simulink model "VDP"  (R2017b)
settings: Solver=FixedStepDiscrete  StartTime=0.0  StopTime=10.0  FixedStep=0.01  RelTol=1e-3  EnableMultiTasking=on
undefined symbols (not defined in the file): ASWTYPE_FALSE, ASWTYPE_TRUE, CcVDP_DiagPermitDelayTi_ms, CcVDP_LeadAcidChgHvOnTi_ms, Enum_ISPNetWkUpSt, VDP0B5_RUNTIME_MS, VDP2A3_RUNTIME_MS, VDP_CONST18000_NUMB, VDP_CONST2080_NUMB, VDP_CONST6000_NUMB
libraries: AIWAYS_Powertrain_BMS_lib x35

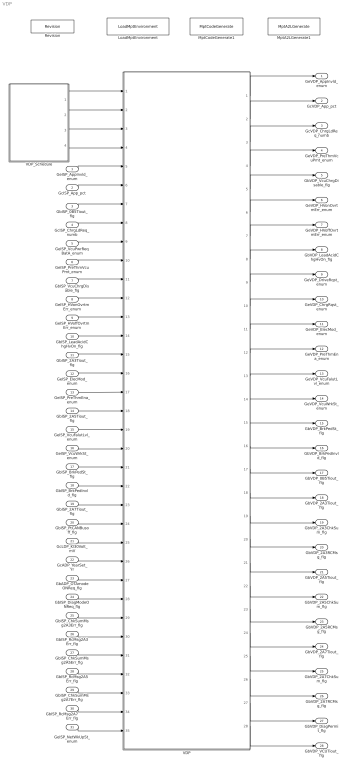
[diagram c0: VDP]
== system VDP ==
  GeISP_AppInvld_enum : Inport
  GcISP_App_pct : Inport  Port=2
  GbISP_0B5Tiout_flg : Inport  Port=3
  GcISP_ChrgLdReq_numb : Inport  Port=4
  GeISP_VcuPwrReqBatA_enum : Inport  Port=5
  GeISP_PreThmVcuPmt_enum : Inport  Port=6
  GbISP_VcuChrgDisable_flg : Inport  Port=7
  GeISP_HVonOvrtmErr_enum : Inport  Port=8
  GeISP_HVoffOvrtmErr_enum : Inport  Port=9
  GbISP_LeadAcidChgHvOn_flg : Inport  Port=10
  GbISP_2A3Tiout_flg : Inport  Port=11
  GeISP_ElecMod_enum : Inport  Port=12
  GeISP_PreThmEna_enum : Inport  Port=13
  GbISP_2A5Tiout_flg : Inport  Port=14
  GeISP_VcuFalutLvl_enum : Inport  Port=15
  GeISP_VcuWrkSt_enum : Inport  Port=16
  GbISP_BrkPedSt_flg : Inport  Port=17
  GbISP_BrkPedInvld_flg : Inport  Port=18
  GbISP_2A7Tiout_flg : Inport  Port=19
  GbISP_PtCANBusoff_flg : Inport  Port=20
  GcLDP_Kl30Volt_mV : Inport  Port=21
  GcADP_YearSet_Yr : Inport  Port=22
  GbADP_OTAmodeONReq_flg : Inport  Port=23
  GbISP_DiagModeONReq_flg : Inport  Port=24
  GbISP_ChkSumMsg2A3Err_flg : Inport  Port=25
  GbISP_RcMsg2A3Err_flg : Inport  Port=26
  GbISP_ChkSumMsg2A5Err_flg : Inport  Port=27
  GbISP_RcMsg2A5Err_flg : Inport  Port=28
  GbISP_ChkSumMsg2A7Err_flg : Inport  Port=29
  GbISP_RcMsg2A7Err_flg : Inport  Port=30
  GeISP_NetWkUpSt_enum : Inport  Port=31
  LoadMptEnvironment : AIWAYS_Powertrain_BMS_lib/Config/LoadMptEnvironment  ProjectName=Comm  SuppierID=NewPlatformUAES
  MptA2LGenerate1 : AIWAYS_Powertrain_BMS_lib/Config/MptA2LGenerate  SystemSampleTime=-1
  MptCodeGenerate1 : AIWAYS_Powertrain_BMS_lib/Config/MptCodeGenerate  SystemSampleTime=-1
  Revision : AIWAYS_Powertrain_BMS_lib/Config/Revision  curVersion='M104C104'  newVersion='M104C104'
  VDP : Subsystem
  VDP_Schedule : Stateflow chart  TreatAsAtomicUnit=on
  GeVDP_AppInvld_enum : Outport
  GcVDP_App_pct : Outport  Port=2
  GcVDP_ChrgLdReq_numb : Outport  Port=3
  GeVDP_PreThmVcuPmt_enum : Outport  Port=4
  GbVDP_VcuChrgDisable_flg : Outport  Port=5
  GeVDP_HVonOvrtmErr_enum : Outport  Port=6
  GeVDP_HVoffOvrtmErr_enum : Outport  Port=7
  GbVDP_LeadAcidChgHvOn_flg : Outport  Port=8
  GeVDP_DriveRqst_enum : Outport  Port=9
  GeVDP_ChrgRqst_enum : Outport  Port=10
  GeVDP_ElecMod_enum : Outport  Port=11
  GeVDP_PreThmEna_enum : Outport  Port=12
  GeVDP_VcuFalutLvl_enum : Outport  Port=13
  GeVDP_VcuWrkSt_enum : Outport  Port=14
  GbVDP_BrkPedSt_flg : Outport  Port=15
  GbVDP_BrkPedInvld_flg : Outport  Port=16
  GbVDP_0B5Tiout_flg : Outport  Port=17
  GbVDP_2A3Tiout_flg : Outport  Port=18
  GbVDP_2A3ChkSum_flg : Outport  Port=19
  GbVDP_2A3RCMsg_flg : Outport  Port=20
  GbVDP_2A5Tiout_flg : Outport  Port=21
  GbVDP_2A5ChkSum_flg : Outport  Port=22
  GbVDP_2A5RCMsg_flg : Outport  Port=23
  GbVDP_2A7Tiout_flg : Outport  Port=24
  GbVDP_2A7ChkSum_flg : Outport  Port=25
  GbVDP_2A7RCMsg_flg : Outport  Port=26
  GbVDP_DiagPermit_flg : Outport  Port=27
  GbVDP_VCUTiout_flg : Outport  Port=28
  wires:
  GeISP_AppInvld_enum/1 -> VDP/5(GeISP_AppInvld_enum)
  GcISP_App_pct/1 -> VDP/6(GcISP_App_pct)
  GbISP_0B5Tiout_flg/1 -> VDP/7(GbISP_0B5Tiout_flg)
  GcISP_ChrgLdReq_numb/1 -> VDP/8(GcISP_ChrgLdReq_numb)
  GeISP_VcuPwrReqBatA_enum/1 -> VDP/9(GeISP_VcuPwrReqBatA_enum)
  GeISP_PreThmVcuPmt_enum/1 -> VDP/10(GeISP_PreThmVcuPmt_enum)
  GbISP_VcuChrgDisable_flg/1 -> VDP/11(GbISP_VcuChrgDisable_flg)
  GeISP_HVonOvrtmErr_enum/1 -> VDP/12(GeISP_HVonOvrtmErr_enum)
  GeISP_HVoffOvrtmErr_enum/1 -> VDP/13(GeISP_HVoffOvrtmErr_enum)
  GbISP_LeadAcidChgHvOn_flg/1 -> VDP/14(GbISP_LeadAcidChgHvOn_flg)
  GbISP_2A3Tiout_flg/1 -> VDP/15(GbISP_2A3Tiout_flg)
  GeISP_ElecMod_enum/1 -> VDP/16(GeISP_ElecMod_enum)
  GeISP_PreThmEna_enum/1 -> VDP/17(GeISP_PreThmEna_enum)
  GbISP_2A5Tiout_flg/1 -> VDP/18(GbISP_2A5Tiout_flg)
  GeISP_VcuFalutLvl_enum/1 -> VDP/19(GeISP_VcuFalutLvl_enum)
  GeISP_VcuWrkSt_enum/1 -> VDP/20(GeISP_VcuWrkSt_enum)
  GbISP_BrkPedSt_flg/1 -> VDP/21(GbISP_BrkPedSt_flg)
  GbISP_BrkPedInvld_flg/1 -> VDP/22(GbISP_BrkPedInvld_flg)
  GbISP_2A7Tiout_flg/1 -> VDP/23(GbISP_2A7Tiout_flg)
  VDP/1(GeVDP_AppInvld_enum) -> GeVDP_AppInvld_enum/1
  VDP/2(GcVDP_App_pct) -> GcVDP_App_pct/1
  VDP/3(GcVDP_ChrgLdReq_numb) -> GcVDP_ChrgLdReq_numb/1
  VDP/4(GeVDP_PreThmVcuPmt_enum) -> GeVDP_PreThmVcuPmt_enum/1
  VDP/5(GbVDP_VcuChrgDisable_flg) -> GbVDP_VcuChrgDisable_flg/1
  VDP/6(GeVDP_HVonOvrtmErr_enum) -> GeVDP_HVonOvrtmErr_enum/1
  VDP/7(GeVDP_HVoffOvrtmErr_enum) -> GeVDP_HVoffOvrtmErr_enum/1
  VDP/8(GbVDP_LeadAcidChgHvOn_flg) -> GbVDP_LeadAcidChgHvOn_flg/1
  VDP/9(GeVDP_DriveRqst_enum) -> GeVDP_DriveRqst_enum/1
  VDP/10(GeVDP_ChrgRqst_enum) -> GeVDP_ChrgRqst_enum/1
  VDP/11(GeVDP_ElecMod_enum) -> GeVDP_ElecMod_enum/1
  VDP/12(GeVDP_PreThmEna_enum) -> GeVDP_PreThmEna_enum/1
  VDP/13(GeVDP_VcuFalutLvl_enum) -> GeVDP_VcuFalutLvl_enum/1
  VDP/14(GeVDP_VcuWrkSt_enum) -> GeVDP_VcuWrkSt_enum/1
  VDP/15(GbVDP_BrkPedSt_flg) -> GbVDP_BrkPedSt_flg/1
  VDP/16(GbVDP_BrkPedInvld_flg) -> GbVDP_BrkPedInvld_flg/1
  GbISP_DiagModeONReq_flg/1 -> VDP/28(GbISP_DiagModeONReq_flg)
  GcLDP_Kl30Volt_mV/1 -> VDP/25(GcLDP_Kl30Volt_mV)
  GbADP_OTAmodeONReq_flg/1 -> VDP/27(GbADP_OTAmodeONReq_flg)
  GcADP_YearSet_Yr/1 -> VDP/26(GcADP_YearSet_Yr)
  GbISP_PtCANBusoff_flg/1 -> VDP/24(GbISP_PtCANBusoff_flg)
  GbISP_ChkSumMsg2A3Err_flg/1 -> VDP/29(GbISP_ChkSumMsg2A3Err_flg)
  GbISP_RcMsg2A3Err_flg/1 -> VDP/30(GbISP_RcMsg2A3Err_flg)
  GbISP_RcMsg2A5Err_flg/1 -> VDP/32(GbISP_RcMsg2A5Err_flg)
  GbISP_ChkSumMsg2A5Err_flg/1 -> VDP/31(GbISP_ChkSumMsg2A5Err_flg)
  GbISP_RcMsg2A7Err_flg/1 -> VDP/34(GbISP_RcMsg2A7Err_flg)
  GbISP_ChkSumMsg2A7Err_flg/1 -> VDP/33(GbISP_ChkSumMsg2A7Err_flg)
  VDP/17(GbVDP_0B5Tiout_flg) -> GbVDP_0B5Tiout_flg/1
  VDP/20(GbVDP_2A3RCMsg_flg) -> GbVDP_2A3RCMsg_flg/1
  VDP/18(GbVDP_2A3Tiout_flg) -> GbVDP_2A3Tiout_flg/1
  VDP/19(GbVDP_2A3ChkSum_flg) -> GbVDP_2A3ChkSum_flg/1
  VDP/23(GbVDP_2A5RCMsg_flg) -> GbVDP_2A5RCMsg_flg/1
  VDP/21(GbVDP_2A5Tiout_flg) -> GbVDP_2A5Tiout_flg/1
  VDP/22(GbVDP_2A5ChkSum_flg) -> GbVDP_2A5ChkSum_flg/1
  VDP/25(GbVDP_2A7ChkSum_flg) -> GbVDP_2A7ChkSum_flg/1
  VDP/24(GbVDP_2A7Tiout_flg) -> GbVDP_2A7Tiout_flg/1
  VDP/26(GbVDP_2A7RCMsg_flg) -> GbVDP_2A7RCMsg_flg/1
  VDP/27(GbVDP_DiagPermit_flg) -> GbVDP_DiagPermit_flg/1
  VDP/28(GbVDP_VCUTiout_flg) -> GbVDP_VCUTiout_flg/1
  GeISP_NetWkUpSt_enum/1 -> VDP/35(GeISP_NetWkUpSt_enum)
  VDP_Schedule/3(VDP_2A5_100ms()) -> VDP/3(VDP_2A5_100ms)
  VDP_Schedule/2(VDP_2A3_10ms()) -> VDP/2(VDP_2A3_10ms)
  VDP_Schedule/1(VDP_0B5_10ms()) -> VDP/1(VDP_0B5_10ms)
  VDP_Schedule/4(VDP_2A7_100ms()) -> VDP/4(VDP_2A7_100ms)

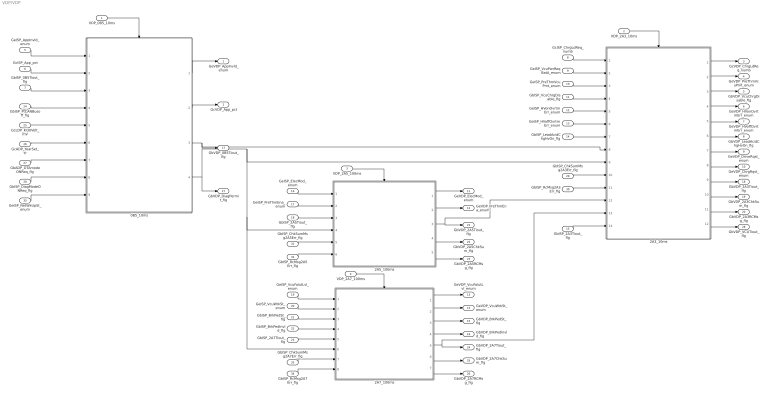
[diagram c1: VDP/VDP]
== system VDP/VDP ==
  VDP_0B5_10ms : Inport
  VDP_2A3_10ms : Inport  Port=2
  VDP_2A5_100ms : Inport  Port=3
  VDP_2A7_100ms : Inport  Port=4
  GeISP_AppInvld_enum : Inport  Port=5
  GcISP_App_pct : Inport  Port=6
  GbISP_0B5Tiout_flg : Inport  Port=7
  GcISP_ChrgLdReq_numb : Inport  Port=8
  GeISP_VcuPwrReqBatA_enum : Inport  Port=9
  GeISP_PreThmVcuPmt_enum : Inport  Port=10
  GbISP_VcuChrgDisable_flg : Inport  Port=11
  GeISP_HVonOvrtmErr_enum : Inport  Port=12
  GeISP_HVoffOvrtmErr_enum : Inport  Port=13
  GbISP_LeadAcidChgHvOn_flg : Inport  Port=14
  GbISP_2A3Tiout_flg : Inport  Port=15
  GeISP_ElecMod_enum : Inport  Port=16
  GeISP_PreThmEna_enum : Inport  Port=17
  GbISP_2A5Tiout_flg : Inport  Port=18
  GeISP_VcuFalutLvl_enum : Inport  Port=19
  GeISP_VcuWrkSt_enum : Inport  Port=20
  GbISP_BrkPedSt_flg : Inport  Port=21
  GbISP_BrkPedInvld_flg : Inport  Port=22
  GbISP_2A7Tiout_flg : Inport  Port=23
  GbISP_PtCANBusoff_flg : Inport  Port=24
  GcLDP_Kl30Volt_mV : Inport  Port=25
  GcADP_YearSet_Yr : Inport  Port=26
  GbADP_OTAmodeONReq_flg : Inport  Port=27
  GbISP_DiagModeONReq_flg : Inport  Port=28
  GbISP_ChkSumMsg2A3Err_flg : Inport  Port=29
  GbISP_RcMsg2A3Err_flg : Inport  Port=30
  GbISP_ChkSumMsg2A5Err_flg : Inport  Port=31
  GbISP_RcMsg2A5Err_flg : Inport  Port=32
  GbISP_ChkSumMsg2A7Err_flg : Inport  Port=33
  GbISP_RcMsg2A7Err_flg : Inport  Port=34
  GeISP_NetWkUpSt_enum : Inport  Port=35
  0B5_10ms : Subsystem
  2A3_10ms : Subsystem
  2A5_100ms : Subsystem
  2A7_100ms : Subsystem
  GeVDP_AppInvld_enum : Outport
  GcVDP_App_pct : Outport  Port=2
  GcVDP_ChrgLdReq_numb : Outport  Port=3
  GeVDP_PreThmVcuPmt_enum : Outport  Port=4
  GbVDP_VcuChrgDisable_flg : Outport  Port=5
  GeVDP_HVonOvrtmErr_enum : Outport  Port=6
  GeVDP_HVoffOvrtmErr_enum : Outport  Port=7
  GbVDP_LeadAcidChgHvOn_flg : Outport  Port=8
  GeVDP_DriveRqst_enum : Outport  Port=9
  GeVDP_ChrgRqst_enum : Outport  Port=10
  GeVDP_ElecMod_enum : Outport  Port=11
  GeVDP_PreThmEna_enum : Outport  Port=12
  GeVDP_VcuFalutLvl_enum : Outport  Port=13
  GeVDP_VcuWrkSt_enum : Outport  Port=14
  GbVDP_BrkPedSt_flg : Outport  Port=15
  GbVDP_BrkPedInvld_flg : Outport  Port=16
  GbVDP_0B5Tiout_flg : Outport  Port=17
  GbVDP_2A3Tiout_flg : Outport  Port=18
  GbVDP_2A3ChkSum_flg : Outport  Port=19
  GbVDP_2A3RCMsg_flg : Outport  Port=20
  GbVDP_2A5Tiout_flg : Outport  Port=21
  GbVDP_2A5ChkSum_flg : Outport  Port=22
  GbVDP_2A5RCMsg_flg : Outport  Port=23
  GbVDP_2A7Tiout_flg : Outport  Port=24
  GbVDP_2A7ChkSum_flg : Outport  Port=25
  GbVDP_2A7RCMsg_flg : Outport  Port=26
  GbVDP_DiagPermit_flg : Outport  Port=27
  GbVDP_VCUTiout_flg : Outport  Port=28
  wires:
  VDP_2A3_10ms/1 -> 2A3_10ms/Trigger
  VDP_2A5_100ms/1 -> 2A5_100ms/Trigger
  VDP_2A7_100ms/1 -> 2A7_100ms/Trigger
  GeISP_AppInvld_enum/1 -> 0B5_10ms/1(GeISP_AppInvld_enum)
  GcISP_App_pct/1 -> 0B5_10ms/2(GcISP_App_pct)
  GbISP_0B5Tiout_flg/1 -> 0B5_10ms/3(GbISP_0B5Tiout_flg)
  0B5_10ms/1(GeVDP_AppInvld_enum) -> GeVDP_AppInvld_enum/1
  0B5_10ms/2(GcVDP_App_pct) -> GcVDP_App_pct/1
  GcISP_ChrgLdReq_numb/1 -> 2A3_10ms/1(GcISP_ChrgLdReq_numb)
  GeISP_VcuPwrReqBatA_enum/1 -> 2A3_10ms/2(GeISP_VcuPwrReqBatA_enum)
  GeISP_PreThmVcuPmt_enum/1 -> 2A3_10ms/3(GeISP_PreThmVcuPmt_enum)
  GbISP_VcuChrgDisable_flg/1 -> 2A3_10ms/4(GbISP_VcuChrgDisable_flg)
  GeISP_HVonOvrtmErr_enum/1 -> 2A3_10ms/5(GeISP_HVonOvrtmErr_enum)
  GeISP_HVoffOvrtmErr_enum/1 -> 2A3_10ms/6(GeISP_HVoffOvrtmErr_enum)
  GbISP_LeadAcidChgHvOn_flg/1 -> 2A3_10ms/7(GbISP_LeadAcidChgHvOn_flg)
  GbISP_2A3Tiout_flg/1 -> 2A3_10ms/14(GbISP_2A3Tiout_flg)
  2A3_10ms/5(GeVDP_HVoffOvrtmErr_enum) -> GeVDP_HVoffOvrtmErr_enum/1
  2A3_10ms/4(GeVDP_HVonOvrtmErr_enum) -> GeVDP_HVonOvrtmErr_enum/1
  2A3_10ms/6(GbVDP_LeadAcidChgHvOn_flg) -> GbVDP_LeadAcidChgHvOn_flg/1
  2A3_10ms/3(GbVDP_VcuChrgDisable_flg) -> GbVDP_VcuChrgDisable_flg/1
  2A3_10ms/2(GeVDP_PreThmVcuPmt_enum) -> GeVDP_PreThmVcuPmt_enum/1
  2A3_10ms/1(GcVDP_ChrgLdReq_numb) -> GcVDP_ChrgLdReq_numb/1
  2A3_10ms/7(GeVDP_DriveRqst_enum) -> GeVDP_DriveRqst_enum/1
  2A3_10ms/8(GeVDP_ChrgRqst_enum) -> GeVDP_ChrgRqst_enum/1
  GeISP_ElecMod_enum/1 -> 2A5_100ms/1(GeISP_ElecMod_enum)
  GeISP_PreThmEna_enum/1 -> 2A5_100ms/2(GeISP_PreThmEna_enum)
  GbISP_2A5Tiout_flg/1 -> 2A5_100ms/3(GbISP_2A5Tiout_flg)
  2A5_100ms/1(GeVDP_ElecMod_enum) -> GeVDP_ElecMod_enum/1
  2A5_100ms/2(GeVDP_PreThmEna_enum) -> GeVDP_PreThmEna_enum/1
  GeISP_VcuFalutLvl_enum/1 -> 2A7_100ms/1(GeISP_VcuFalutLvl_enum)
  GeISP_VcuWrkSt_enum/1 -> 2A7_100ms/2(GeISP_VcuWrkSt_enum)
  GbISP_BrkPedSt_flg/1 -> 2A7_100ms/3(GbISP_BrkPedSt_flg)
  GbISP_BrkPedInvld_flg/1 -> 2A7_100ms/4(GbISP_BrkPedInvld_flg)
  GbISP_2A7Tiout_flg/1 -> 2A7_100ms/5(GbISP_2A7Tiout_flg)
  2A7_100ms/1(GeVDP_VcuFalutLvl_enum) -> GeVDP_VcuFalutLvl_enum/1
  2A7_100ms/2(GeVDP_VcuWrkSt_enum) -> GeVDP_VcuWrkSt_enum/1
  2A7_100ms/3(GbVDP_BrkPedSt_flg) -> GbVDP_BrkPedSt_flg/1
  2A7_100ms/4(GbVDP_BrkPedInvld_flg) -> GbVDP_BrkPedInvld_flg/1
  0B5_10ms/3(GbVDP_0B5Tiout_flg) -> GbVDP_0B5Tiout_flg/1, 2A3_10ms/8(GbVDP_0B5Tiout_flg)
  GbISP_ChkSumMsg2A3Err_flg/1 -> 2A3_10ms/10(GbISP_ChkSumMsg2A3Err_flg)
  GbISP_RcMsg2A3Err_flg/1 -> 2A3_10ms/11(GbISP_RcMsg2A3Err_flg)
  2A3_10ms/9(GbVDP_2A3Tiout_flg) -> GbVDP_2A3Tiout_flg/1
  2A3_10ms/10(GbVDP_2A3ChkSum_flg) -> GbVDP_2A3ChkSum_flg/1
  2A3_10ms/11(GbVDP_2A3RCMsg_flg) -> GbVDP_2A3RCMsg_flg/1
  GbISP_ChkSumMsg2A5Err_flg/1 -> 2A5_100ms/5(GbISP_ChkSumMsg2A5Err_flg)
  GbISP_RcMsg2A5Err_flg/1 -> 2A5_100ms/6(GbISP_RcMsg2A5Err_flg)
  2A5_100ms/5(GbVDP_2A5RCMsg_flg) -> GbVDP_2A5RCMsg_flg/1
  2A5_100ms/3(GbVDP_2A5Tiout_flg) -> GbVDP_2A5Tiout_flg/1, 2A3_10ms/12(GbVDP_2A5Tiout_flg)
  2A5_100ms/4(GbVDP_2A5ChkSum_flg) -> GbVDP_2A5ChkSum_flg/1
  GbISP_RcMsg2A7Err_flg/1 -> 2A7_100ms/8(GbISP_RcMsg2A7Err_flg)
  GbISP_ChkSumMsg2A7Err_flg/1 -> 2A7_100ms/7(GbISP_ChkSumMsg2A7Err_flg)
  2A7_100ms/7(GbVDP_2A7RCMsg_flg) -> GbVDP_2A7RCMsg_flg/1
  2A7_100ms/5(GbVDP_2A7Tiout_flg) -> GbVDP_2A7Tiout_flg/1, 2A3_10ms/13(GbVDP_2A7Tiout_flg)
  2A7_100ms/6(GbVDP_2A7ChkSum_flg) -> GbVDP_2A7ChkSum_flg/1
  GcLDP_Kl30Volt_mV/1 -> 0B5_10ms/5(GcLDP_Kl30Volt_mV)
  GcADP_YearSet_Yr/1 -> 0B5_10ms/6(GcADP_YearSet_Yr)
  GbADP_OTAmodeONReq_flg/1 -> 0B5_10ms/7(GbADP_OTAmodeONReq_flg)
  GbISP_DiagModeONReq_flg/1 -> 0B5_10ms/8(GbISP_DiagModeONReq_flg)
  0B5_10ms/4(GbVDP_DiagPermit_flg) -> 2A7_100ms/6(GbVDP_DiagPermit_flg), 2A5_100ms/4(GbVDP_DiagPermit_flg), 2A3_10ms/9(GbVDP_DiagPermit_flg), GbVDP_DiagPermit_flg/1
  VDP_0B5_10ms/1 -> 0B5_10ms/Trigger
  GbISP_PtCANBusoff_flg/1 -> 0B5_10ms/4(GbISP_PtCANBusoff_flg)
  2A3_10ms/12(GbVDP_VCUTiout_flg) -> GbVDP_VCUTiout_flg/1
  GeISP_NetWkUpSt_enum/1 -> 0B5_10ms/9(GeISP_NetWkUpSt_enum)

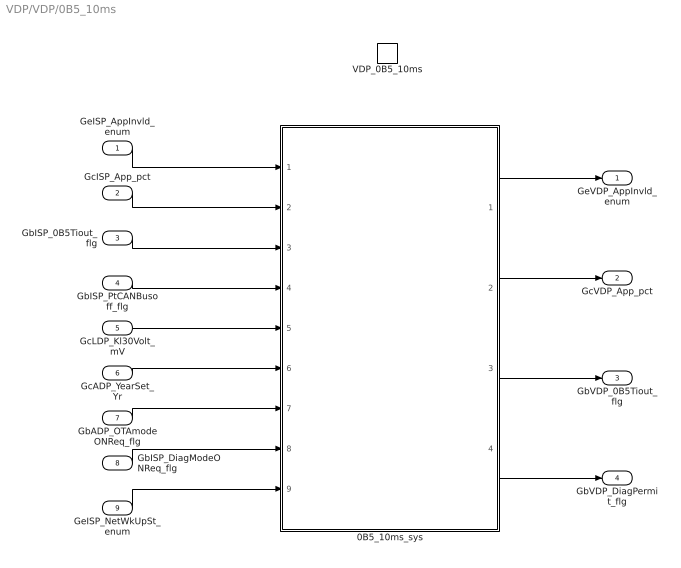
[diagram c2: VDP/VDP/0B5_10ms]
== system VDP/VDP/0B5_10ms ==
  GeISP_AppInvld_enum : Inport
  GcISP_App_pct : Inport  Port=2
  GbISP_0B5Tiout_flg : Inport  Port=3
  GbISP_PtCANBusoff_flg : Inport  Port=4
  GcLDP_Kl30Volt_mV : Inport  Port=5
  GcADP_YearSet_Yr : Inport  Port=6
  GbADP_OTAmodeONReq_flg : Inport  Port=7
  GbISP_DiagModeONReq_flg : Inport  Port=8
  GeISP_NetWkUpSt_enum : Inport  Port=9
  VDP_0B5_10ms : TriggerPort  TriggerType=function-call  VariantControl=(inherit)
  0B5_10ms_sys : Subsystem
  GeVDP_AppInvld_enum : Outport
  GcVDP_App_pct : Outport  Port=2
  GbVDP_0B5Tiout_flg : Outport  Port=3
  GbVDP_DiagPermit_flg : Outport  Port=4
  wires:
  GeISP_AppInvld_enum/1 -> 0B5_10ms_sys/1(GeISP_AppInvld_enum)
  GcISP_App_pct/1 -> 0B5_10ms_sys/2(GcISP_App_pct)
  GbISP_0B5Tiout_flg/1 -> 0B5_10ms_sys/3(GbISP_0B5Tiout_flg)
  0B5_10ms_sys/1(GeVDP_AppInvld_enum) -> GeVDP_AppInvld_enum/1
  0B5_10ms_sys/2(GcVDP_App_pct) -> GcVDP_App_pct/1
  0B5_10ms_sys/3(GbVDP_0B5Tiout_flg) -> GbVDP_0B5Tiout_flg/1
  GbISP_PtCANBusoff_flg/1 -> 0B5_10ms_sys/4(GbISP_PtCANBusoff_flg)
  GbISP_DiagModeONReq_flg/1 -> 0B5_10ms_sys/8(GbISP_DiagModeONReq_flg)
  GcADP_YearSet_Yr/1 -> 0B5_10ms_sys/6(GcADP_YearSet_Yr)
  GcLDP_Kl30Volt_mV/1 -> 0B5_10ms_sys/5(GcLDP_Kl30Volt_mV)
  GbADP_OTAmodeONReq_flg/1 -> 0B5_10ms_sys/7(GbADP_OTAmodeONReq_flg)
  0B5_10ms_sys/4(GbVDP_DiagPermit_flg) -> GbVDP_DiagPermit_flg/1
  GeISP_NetWkUpSt_enum/1 -> 0B5_10ms_sys/9(GeISP_NetWkUpSt_enum)

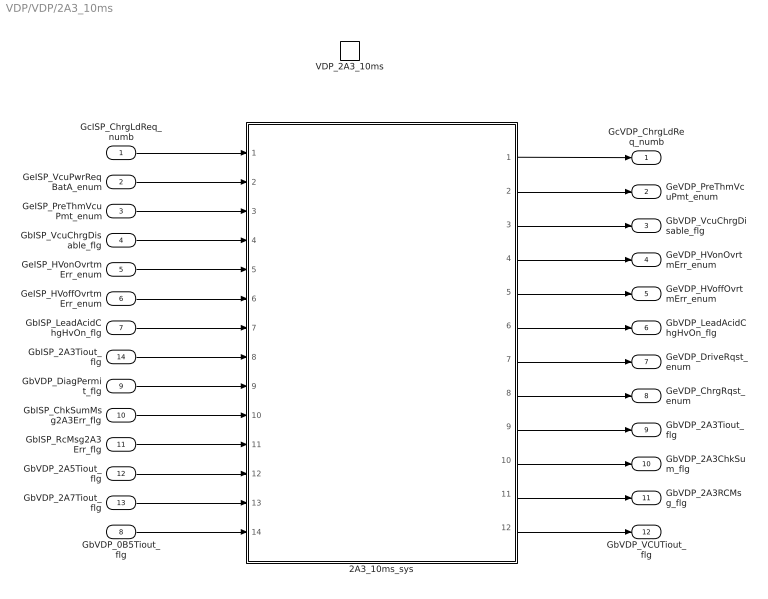
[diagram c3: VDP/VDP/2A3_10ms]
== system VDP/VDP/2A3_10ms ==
  GcISP_ChrgLdReq_numb : Inport
  GeISP_VcuPwrReqBatA_enum : Inport  Port=2
  GeISP_PreThmVcuPmt_enum : Inport  Port=3
  GbISP_VcuChrgDisable_flg : Inport  Port=4
  GeISP_HVonOvrtmErr_enum : Inport  Port=5
  GeISP_HVoffOvrtmErr_enum : Inport  Port=6
  GbISP_LeadAcidChgHvOn_flg : Inport  Port=7
  GbVDP_0B5Tiout_flg : Inport  Port=8
  GbVDP_DiagPermit_flg : Inport  Port=9
  GbISP_ChkSumMsg2A3Err_flg : Inport  Port=10
  GbISP_RcMsg2A3Err_flg : Inport  Port=11
  GbVDP_2A5Tiout_flg : Inport  Port=12
  GbVDP_2A7Tiout_flg : Inport  Port=13
  GbISP_2A3Tiout_flg : Inport  Port=14
  VDP_2A3_10ms : TriggerPort  TriggerType=function-call  VariantControl=(inherit)
  2A3_10ms_sys : Subsystem
  GcVDP_ChrgLdReq_numb : Outport
  GeVDP_PreThmVcuPmt_enum : Outport  Port=2
  GbVDP_VcuChrgDisable_flg : Outport  Port=3
  GeVDP_HVonOvrtmErr_enum : Outport  Port=4
  GeVDP_HVoffOvrtmErr_enum : Outport  Port=5
  GbVDP_LeadAcidChgHvOn_flg : Outport  Port=6
  GeVDP_DriveRqst_enum : Outport  Port=7
  GeVDP_ChrgRqst_enum : Outport  Port=8
  GbVDP_2A3Tiout_flg : Outport  Port=9
  GbVDP_2A3ChkSum_flg : Outport  Port=10
  GbVDP_2A3RCMsg_flg : Outport  Port=11
  GbVDP_VCUTiout_flg : Outport  Port=12
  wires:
  GcISP_ChrgLdReq_numb/1 -> 2A3_10ms_sys/1(GcISP_ChrgLdReq_numb)
  GeISP_VcuPwrReqBatA_enum/1 -> 2A3_10ms_sys/2(GeISP_VcuPwrReqBatA_enum)
  GeISP_PreThmVcuPmt_enum/1 -> 2A3_10ms_sys/3(GeISP_PreThmVcuPmt_enum)
  GbISP_VcuChrgDisable_flg/1 -> 2A3_10ms_sys/4(GbISP_VcuChrgDisable_flg)
  GeISP_HVonOvrtmErr_enum/1 -> 2A3_10ms_sys/5(GeISP_HVonOvrtmErr_enum)
  GeISP_HVoffOvrtmErr_enum/1 -> 2A3_10ms_sys/6(GeISP_HVoffOvrtmErr_enum)
  GbISP_LeadAcidChgHvOn_flg/1 -> 2A3_10ms_sys/7(GbISP_LeadAcidChgHvOn_flg)
  GbISP_2A3Tiout_flg/1 -> 2A3_10ms_sys/8(GbISP_2A3Tiout_flg)
  2A3_10ms_sys/1(GcVDP_ChrgLdReq_numb) -> GcVDP_ChrgLdReq_numb/1
  2A3_10ms_sys/2(GeVDP_PreThmVcuPmt_enum) -> GeVDP_PreThmVcuPmt_enum/1
  2A3_10ms_sys/3(GbVDP_VcuChrgDisable_flg) -> GbVDP_VcuChrgDisable_flg/1
  2A3_10ms_sys/4(GeVDP_HVonOvrtmErr_enum) -> GeVDP_HVonOvrtmErr_enum/1
  2A3_10ms_sys/5(GeVDP_HVoffOvrtmErr_enum) -> GeVDP_HVoffOvrtmErr_enum/1
  2A3_10ms_sys/6(GbVDP_LeadAcidChgHvOn_flg) -> GbVDP_LeadAcidChgHvOn_flg/1
  2A3_10ms_sys/7(GeVDP_DriveRqst_enum) -> GeVDP_DriveRqst_enum/1
  2A3_10ms_sys/8(GeVDP_ChrgRqst_enum) -> GeVDP_ChrgRqst_enum/1
  GbVDP_DiagPermit_flg/1 -> 2A3_10ms_sys/9(GbVDP_DiagPermit_flg)
  2A3_10ms_sys/9(GbVDP_2A3Tiout_flg) -> GbVDP_2A3Tiout_flg/1
  2A3_10ms_sys/10(GbVDP_2A3ChkSum_flg) -> GbVDP_2A3ChkSum_flg/1
  2A3_10ms_sys/11(GbVDP_2A3RCMsg_flg) -> GbVDP_2A3RCMsg_flg/1
  GbISP_ChkSumMsg2A3Err_flg/1 -> 2A3_10ms_sys/10(GbISP_ChkSumMsg2A3Err_flg)
  GbISP_RcMsg2A3Err_flg/1 -> 2A3_10ms_sys/11(GbISP_RcMsg2A3Err_flg)
  2A3_10ms_sys/12(GbVDP_VCUTiout_flg) -> GbVDP_VCUTiout_flg/1
  GbVDP_2A5Tiout_flg/1 -> 2A3_10ms_sys/12(GbVDP_2A5Tiout_flg)
  GbVDP_2A7Tiout_flg/1 -> 2A3_10ms_sys/13(GbVDP_2A7Tiout_flg)
  GbVDP_0B5Tiout_flg/1 -> 2A3_10ms_sys/14(GbVDP_0B5Tiout_flg)

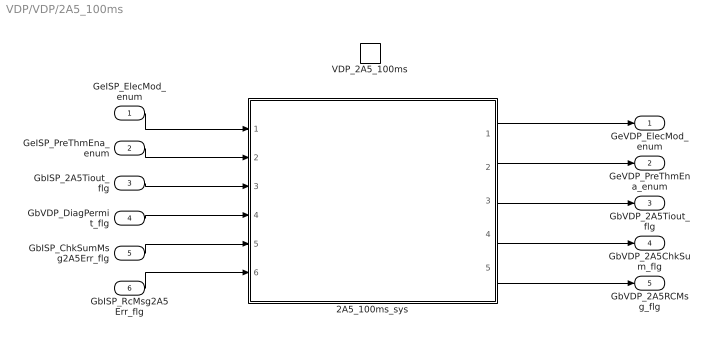
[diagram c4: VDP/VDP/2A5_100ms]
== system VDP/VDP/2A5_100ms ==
  GeISP_ElecMod_enum : Inport
  GeISP_PreThmEna_enum : Inport  Port=2
  GbISP_2A5Tiout_flg : Inport  Port=3
  GbVDP_DiagPermit_flg : Inport  Port=4
  GbISP_ChkSumMsg2A5Err_flg : Inport  Port=5
  GbISP_RcMsg2A5Err_flg : Inport  Port=6
  VDP_2A5_100ms : TriggerPort  TriggerType=function-call  VariantControl=(inherit)
  2A5_100ms_sys : Subsystem
  GeVDP_ElecMod_enum : Outport
  GeVDP_PreThmEna_enum : Outport  Port=2
  GbVDP_2A5Tiout_flg : Outport  Port=3
  GbVDP_2A5ChkSum_flg : Outport  Port=4
  GbVDP_2A5RCMsg_flg : Outport  Port=5
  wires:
  GeISP_ElecMod_enum/1 -> 2A5_100ms_sys/1(GeISP_ElecMod_enum)
  GeISP_PreThmEna_enum/1 -> 2A5_100ms_sys/2(GeISP_PreThmEna_enum)
  GbISP_2A5Tiout_flg/1 -> 2A5_100ms_sys/3(GbISP_2A5Tiout_flg)
  2A5_100ms_sys/1(GeVDP_ElecMod_enum) -> GeVDP_ElecMod_enum/1
  2A5_100ms_sys/2(GeVDP_PreThmEna_enum) -> GeVDP_PreThmEna_enum/1
  GbVDP_DiagPermit_flg/1 -> 2A5_100ms_sys/4(GbVDP_DiagPermit_flg)
  2A5_100ms_sys/3(GbVDP_2A5Tiout_flg) -> GbVDP_2A5Tiout_flg/1
  2A5_100ms_sys/4(GbVDP_2A5ChkSum_flg) -> GbVDP_2A5ChkSum_flg/1
  2A5_100ms_sys/5(GbVDP_2A5RCMsg_flg) -> GbVDP_2A5RCMsg_flg/1
  GbISP_ChkSumMsg2A5Err_flg/1 -> 2A5_100ms_sys/5(GbISP_ChkSumMsg2A5Err_flg)
  GbISP_RcMsg2A5Err_flg/1 -> 2A5_100ms_sys/6(GbISP_RcMsg2A5Err_flg)

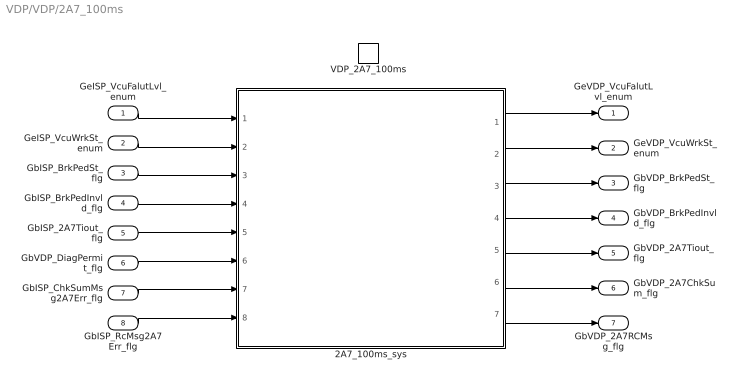
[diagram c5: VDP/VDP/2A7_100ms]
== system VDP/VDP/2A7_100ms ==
  GeISP_VcuFalutLvl_enum : Inport
  GeISP_VcuWrkSt_enum : Inport  Port=2
  GbISP_BrkPedSt_flg : Inport  Port=3
  GbISP_BrkPedInvld_flg : Inport  Port=4
  GbISP_2A7Tiout_flg : Inport  Port=5
  GbVDP_DiagPermit_flg : Inport  Port=6
  GbISP_ChkSumMsg2A7Err_flg : Inport  Port=7
  GbISP_RcMsg2A7Err_flg : Inport  Port=8
  VDP_2A7_100ms : TriggerPort  TriggerType=function-call  VariantControl=(inherit)
  2A7_100ms_sys : Subsystem
  GeVDP_VcuFalutLvl_enum : Outport
  GeVDP_VcuWrkSt_enum : Outport  Port=2
  GbVDP_BrkPedSt_flg : Outport  Port=3
  GbVDP_BrkPedInvld_flg : Outport  Port=4
  GbVDP_2A7Tiout_flg : Outport  Port=5
  GbVDP_2A7ChkSum_flg : Outport  Port=6
  GbVDP_2A7RCMsg_flg : Outport  Port=7
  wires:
  GeISP_VcuFalutLvl_enum/1 -> 2A7_100ms_sys/1(GeISP_VcuFalutLvl_enum)
  GeISP_VcuWrkSt_enum/1 -> 2A7_100ms_sys/2(GeISP_VcuWrkSt_enum)
  GbISP_BrkPedSt_flg/1 -> 2A7_100ms_sys/3(GbISP_BrkPedSt_flg)
  GbISP_BrkPedInvld_flg/1 -> 2A7_100ms_sys/4(GbISP_BrkPedInvld_flg)
  GbISP_2A7Tiout_flg/1 -> 2A7_100ms_sys/5(GbISP_2A7Tiout_flg)
  2A7_100ms_sys/1(GeVDP_VcuFalutLvl_enum) -> GeVDP_VcuFalutLvl_enum/1
  2A7_100ms_sys/2(GeVDP_VcuWrkSt_enum) -> GeVDP_VcuWrkSt_enum/1
  2A7_100ms_sys/3(GbVDP_BrkPedSt_flg) -> GbVDP_BrkPedSt_flg/1
  2A7_100ms_sys/4(GbVDP_BrkPedInvld_flg) -> GbVDP_BrkPedInvld_flg/1
  GbVDP_DiagPermit_flg/1 -> 2A7_100ms_sys/6(GbVDP_DiagPermit_flg)
  GbISP_ChkSumMsg2A7Err_flg/1 -> 2A7_100ms_sys/7(GbISP_ChkSumMsg2A7Err_flg)
  GbISP_RcMsg2A7Err_flg/1 -> 2A7_100ms_sys/8(GbISP_RcMsg2A7Err_flg)
  2A7_100ms_sys/5(GbVDP_2A7Tiout_flg) -> GbVDP_2A7Tiout_flg/1
  2A7_100ms_sys/7(GbVDP_2A7RCMsg_flg) -> GbVDP_2A7RCMsg_flg/1
  2A7_100ms_sys/6(GbVDP_2A7ChkSum_flg) -> GbVDP_2A7ChkSum_flg/1

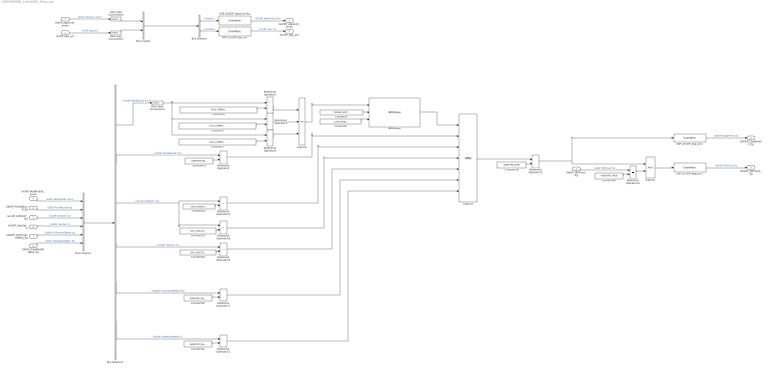
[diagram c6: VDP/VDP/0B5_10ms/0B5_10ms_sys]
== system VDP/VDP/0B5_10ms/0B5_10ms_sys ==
  GeISP_AppInvld_enum : Inport
  GcISP_App_pct : Inport  Port=2
  GbISP_0B5Tiout_flg : Inport  Port=3
  GbISP_PtCANBusoff_flg : Inport  Port=4
  GcLDP_Kl30Volt_mV : Inport  Port=5
  GcADP_YearSet_Yr : Inport  Port=6
  GbADP_OTAmodeONReq_flg : Inport  Port=7
  GbISP_DiagModeONReq_flg : Inport  Port=8
  GeISP_NetWkUpSt_enum : Inport  Port=9
  BMSDelay : AIWAYS_Powertrain_BMS_lib/Debounce & Delay/BMSDelay
  Bus Creator : BusCreator  Inputs=2
  Bus Creator1 : BusCreator  Inputs=6
  Bus Selector : BusSelector  OutputSignals=signal1,signal2
  Bus Selector1 : BusSelector  OutputSignals=GeISP_NetWkUpSt_enum,GbISP_PtCANBusoff_flg,GcLDP_Kl30Volt_mV,GcADP_YearSet_Yr,GbADP_OTAmodeONReq_flg,GbISP_DiagModeONReq_flg
  Constant1 : Constant  Value=Enum_ISPNetWkUpSt.Enum_ISPNetWkUpSt_ReadySleep
  Constant14 : Constant  Value=ASWTYPE_TRUE
  Constant15 : Constant  Value=ASWTYPE_FALSE
  Constant17 : Constant  Value=ASWTYPE_FALSE
  Constant18 : Constant  Value=ASWTYPE_TRUE
  Constant2 : Constant  Value=Enum_ISPNetWkUpSt.Enum_ISPNetWkUpSt_NormalOperation
  Constant22 : Constant  Value=VDP_CONST6000_NUMB
  Constant23 : Constant  Value=VDP_CONST18000_NUMB
  Constant24 : Constant  Value=VDP_CONST2080_NUMB
  Constant25 : Constant  Value=ASWTYPE_FALSE
  Constant3 : Constant  Value=Enum_ISPNetWkUpSt.Enum_ISPNetWkUpSt_RepeatMessage
  Constant4 : Constant  Value=CcVDP_DiagPermitDelayTi_ms
  Constant5 : Constant  Value=VDP0B5_RUNTIME_MS
  Data Type Conversion1 : DataTypeConversion
  Data Type Conversion5 : DataTypeConversion
  Data Type Conversion7 : DataTypeConversion
  Logical1 : Logic  Operator=OR  Inputs=3  OutDataTypeStr=boolean
  Logical2 : Logic  OutDataTypeStr=boolean
  Logical3 : Logic  Inputs=7  OutDataTypeStr=boolean
  Relational Operator{1..4,11..14} (8 alike) : RelationalOperator  Operator===  OutDataTypeStr=boolean
  Relational Operator10 : RelationalOperator  Operator=~=  OutDataTypeStr=boolean
  Relational Operator15 : RelationalOperator  Operator=>  OutDataTypeStr=boolean
  Relational Operator16 : RelationalOperator  Operator=<  OutDataTypeStr=boolean
  VDP_GbVDP_AppInvld_flg : AIWAYS_Powertrain_BMS_lib/Signals/OverWrite  OverWrite_Value=CeVDP_AppInvldOvr_enum  OverWrite_flag=CbVDP_AppInvldOvrSwt_flg
  VDP_GcVDP_App_pct : AIWAYS_Powertrain_BMS_lib/Signals/OverWrite  OverWrite_Value=CcVDP_AppOvr_pct  OverWrite_flag=CbVDP_AppOvrSwt_flg
  VDP_GcVDP_App_pct1 : AIWAYS_Powertrain_BMS_lib/Signals/OverWrite  OverWrite_Value=CbVDP_0B5TioutOvr_flg  OverWrite_flag=CbVDP_0B5TioutOvrSwt_flg
  VDP_GcVDP_App_pct2 : AIWAYS_Powertrain_BMS_lib/Signals/OverWrite  OverWrite_Value=CbVDP_DiagPermitOvr_flg  OverWrite_flag=CbVDP_DiagPermitOvrSwt_flg
  GeVDP_AppInvld_enum : Outport
  GcVDP_App_pct : Outport  Port=2
  GbVDP_0B5Tiout_flg : Outport  Port=3
  GbVDP_DiagPermit_flg : Outport  Port=4
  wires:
  Data Type Conversion7/1 -> Bus Creator/2
  GbISP_0B5Tiout_flg/1 -> Relational Operator14/1  "GbISP_0B5Tiout_flg"
  GeISP_AppInvld_enum/1 -> Data Type Conversion5/1  "GeISP_AppInvld_enum"
  GcISP_App_pct/1 -> Data Type Conversion7/1  "GcISP_App_pct"
  Bus Creator/1 -> Bus Selector/1
  Bus Selector/1 -> VDP_GbVDP_AppInvld_flg/1  "<signal1>"
  VDP_GbVDP_AppInvld_flg/1 -> GeVDP_AppInvld_enum/1  "GeVDP_AppInvld_enum"
  Bus Selector/2 -> VDP_GcVDP_App_pct/1  "<signal2>"
  VDP_GcVDP_App_pct/1 -> GcVDP_App_pct/1  "GcVDP_App_pct"
  Data Type Conversion5/1 -> Bus Creator/1
  Constant14/1 -> Relational Operator14/2
  Relational Operator14/1 -> Logical2/2
  Logical2/1 -> VDP_GcVDP_App_pct1/1
  VDP_GcVDP_App_pct1/1 -> GbVDP_0B5Tiout_flg/1  "GbVDP_0B5Tiout_flg"
  Relational Operator15/1 -> Logical3/3
  Constant23/1 -> Relational Operator16/2
  Bus Creator1/1 -> Bus Selector1/1
  Constant17/1 -> Relational Operator2/2
  GbISP_PtCANBusoff_flg/1 -> Bus Creator1/2  "GbISP_PtCANBusoff_flg"
  GcLDP_Kl30Volt_mV/1 -> Bus Creator1/3  "GcLDP_Kl30Volt_mV"
  Constant15/1 -> Relational Operator12/2
  Relational Operator10/1 -> Logical3/5
  Bus Selector1/4 -> Relational Operator10/1  "<GcADP_YearSet_Yr>"
  Bus Selector1/3 -> Relational Operator16/1, Relational Operator15/1  "<GcLDP_Kl30Volt_mV>"
  Relational Operator12/1 -> Logical3/7
  Constant22/1 -> Relational Operator15/2
  BMSDelay/1 -> Logical3/1
  Bus Selector1/6 -> Relational Operator12/1  "<GbISP_DiagModeONReq_flg>"
  Bus Selector1/5 -> Relational Operator11/1  "<GbADP_OTAmodeONReq_flg>"
  Relational Operator16/1 -> Logical3/4
  Constant24/1 -> Relational Operator10/2
  GcADP_YearSet_Yr/1 -> Bus Creator1/4  "GcADP_YearSet_Yr"
  Logical3/1 -> Relational Operator13/1
  Relational Operator13/1 -> VDP_GcVDP_App_pct2/1, Logical2/1
  Relational Operator2/1 -> Logical3/2
  Relational Operator11/1 -> Logical3/6
  Constant18/1 -> Relational Operator13/2
  GbADP_OTAmodeONReq_flg/1 -> Bus Creator1/5  "GbADP_OTAmodeONReq_flg"
  Constant25/1 -> Relational Operator11/2
  GbISP_DiagModeONReq_flg/1 -> Bus Creator1/6  "GbISP_DiagModeONReq_flg"
  Bus Selector1/2 -> Relational Operator2/1  "<GbISP_PtCANBusoff_flg>"
  VDP_GcVDP_App_pct2/1 -> GbVDP_DiagPermit_flg/1  "GbVDP_DiagPermit_flg"
  GeISP_NetWkUpSt_enum/1 -> Bus Creator1/1  "GeISP_NetWkUpSt_enum"
  Data Type Conversion1/1 -> Relational Operator1/1, Relational Operator4/1, Relational Operator3/1
  Constant1/1 -> Relational Operator1/2
  Relational Operator1/1 -> Logical1/1
  Constant2/1 -> Relational Operator3/2
  Constant3/1 -> Relational Operator4/2
  Bus Selector1/1 -> Data Type Conversion1/1  "<GeISP_NetWkUpSt_enum>"
  Relational Operator3/1 -> Logical1/2
  Relational Operator4/1 -> Logical1/3
  Constant5/1 -> BMSDelay/2
  Constant4/1 -> BMSDelay/3
  Logical1/1 -> BMSDelay/1

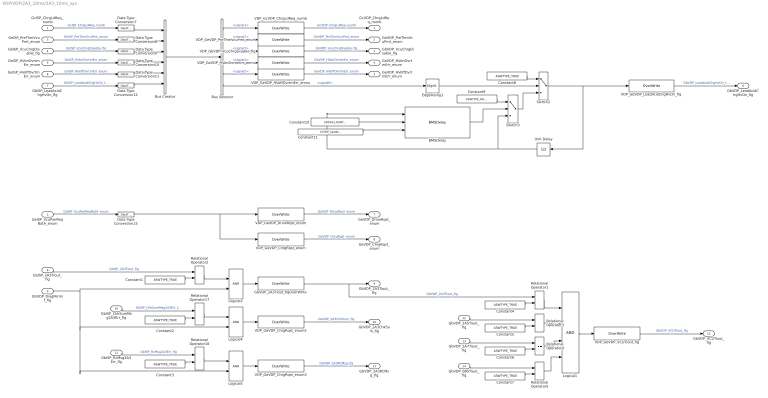
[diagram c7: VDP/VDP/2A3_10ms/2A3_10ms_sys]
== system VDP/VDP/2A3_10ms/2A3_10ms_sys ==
  GcISP_ChrgLdReq_numb : Inport
  GeISP_VcuPwrReqBatA_enum : Inport  Port=2
  GeISP_PreThmVcuPmt_enum : Inport  Port=3
  GbISP_VcuChrgDisable_flg : Inport  Port=4
  GeISP_HVonOvrtmErr_enum : Inport  Port=5
  GeISP_HVoffOvrtmErr_enum : Inport  Port=6
  GbISP_LeadAcidChgHvOn_flg : Inport  Port=7
  GbISP_2A3Tiout_flg : Inport  Port=8
  GbVDP_DiagPermit_flg : Inport  Port=9
  GbISP_ChkSumMsg2A3Err_flg : Inport  Port=10
  GbISP_RcMsg2A3Err_flg : Inport  Port=11
  GbVDP_2A5Tiout_flg : Inport  Port=12
  GbVDP_2A7Tiout_flg : Inport  Port=13
  GbVDP_0B5Tiout_flg : Inport  Port=14
  BMSDelay : AIWAYS_Powertrain_BMS_lib/Debounce & Delay/BMSDelay
  Bus Creator : BusCreator  Inputs=6
  Bus Selector : BusSelector  OutputSignals=signal1,signal2,signal3,signal4,signal5,signal6
  Constant{1..8} (8 alike) : Constant  Value=ASWTYPE_TRUE
  Constant10 : Constant  Value=VDP2A3_RUNTIME_MS
  Constant11 : Constant  Value=CcVDP_LeadAcidChgHvOnTi_ms
  Constant9 : Constant  Value=ASWTYPE_FALSE
  Data Type Conversion{7..12,15} (7 alike) : DataTypeConversion
  EdgeRising1 : AIWAYS_Powertrain_BMS_lib/Logical Operators/EdgeRising
  GbVDP_2A3Tiout_flgOverWrite : AIWAYS_Powertrain_BMS_lib/Signals/OverWrite  OverWrite_Value=CbVDP_2A3TioutOvr_flg  OverWrite_flag=CbVDP_2A3TioutOvrSwt_flg
  Logical1 : Logic  Inputs=4  OutDataTypeStr=boolean
  Logical2 : Logic  OutDataTypeStr=boolean
  Logical4 : Logic  OutDataTypeStr=boolean
  Logical5 : Logic  OutDataTypeStr=boolean
  Relational Operator{1..5,17..18} (7 alike) : RelationalOperator  Operator===  OutDataTypeStr=boolean
  Switch2 : Switch  Criteria=u2 ~= 0
  Switch3 : Switch  Criteria=u2 ~= 0
  Unit Delay : UnitDelay  SampleTime=-1  StateName=StateName
  VDP_GbVDP_LeadAcidChgHvOn_flg : AIWAYS_Powertrain_BMS_lib/Signals/OverWrite  OverWrite_Value=CbVDP_LeadAcidChgHvOnOvr_flg  OverWrite_flag=CbVDP_LeadAcidChgHvOnOvrSwt_flg
  VDP_GbVDP_VCUTiout_flg : AIWAYS_Powertrain_BMS_lib/Signals/OverWrite  OverWrite_Value=CbVDP_VCUTioutOvr_flg  OverWrite_flag=CbVDP_VCUTioutOvrSwt_flg
  VDP_GbVDP_VcuChrgDisable_flg : AIWAYS_Powertrain_BMS_lib/Signals/OverWrite  OverWrite_Value=CbVDP_VcuChrgDisableOvr_flg  OverWrite_flag=CbVDP_VcuChrgDisableOvrSwt_flg
  VDP_GcVDP_ChrgLdReq_numb : AIWAYS_Powertrain_BMS_lib/Signals/OverWrite  OverWrite_Value=CcVDP_ChrgLdReqOvr_numb  OverWrite_flag=CbVDP_ChrgLdReqOvrSwt_flg
  VDP_GeVDP_ChrgRqst_enum : AIWAYS_Powertrain_BMS_lib/Signals/OverWrite  OverWrite_Value=CeVDP_ChrgRqstOvr_enum  OverWrite_flag=CbVDP_ChrgRqstOvrSwt_flg
  VDP_GeVDP_ChrgRqst_enum2 : AIWAYS_Powertrain_BMS_lib/Signals/OverWrite  OverWrite_Value=CbVDP_2A3ChkSumOvr_flg  OverWrite_flag=CbVDP_2A3ChkSumOvrSwt_flg
  VDP_GeVDP_ChrgRqst_enum3 : AIWAYS_Powertrain_BMS_lib/Signals/OverWrite  OverWrite_Value=CbVDP_2A3RCMsgOvr_flg  OverWrite_flag=CbVDP_2A3RCMsgOvrSwt_flg
  VDP_GeVDP_DriveRqst_enum : AIWAYS_Powertrain_BMS_lib/Signals/OverWrite  OverWrite_Value=CeVDP_DriveRqstOvr_enum  OverWrite_flag=CbVDP_DriveRqstOvrSwt_flg
  VDP_GeVDP_HVoffOvrtmErr_enmu : AIWAYS_Powertrain_BMS_lib/Signals/OverWrite  OverWrite_Value=CeVDP_HVoffOvrtmErrOvr_enum  OverWrite_flag=CbVDP_HVoffOvrtmErrOvrSwt_flg
  VDP_GeVDP_HVonOvrtmErr_enmu : AIWAYS_Powertrain_BMS_lib/Signals/OverWrite  OverWrite_Value=CeVDP_HVonOvrtmErrOvr_enum  OverWrite_flag=CbVDP_HVonOvrtmErrOvrSwt_flg
  VDP_GeVDP_PreThmVcuPmt_enum : AIWAYS_Powertrain_BMS_lib/Signals/OverWrite  OverWrite_Value=CeVDP_PreThmVcuPmtOvr_enum  OverWrite_flag=CbVDP_PreThmVcuPmtOvrSwt_flg
  GcVDP_ChrgLdReq_numb : Outport
  GeVDP_PreThmVcuPmt_enum : Outport  Port=2
  GbVDP_VcuChrgDisable_flg : Outport  Port=3
  GeVDP_HVonOvrtmErr_enum : Outport  Port=4
  GeVDP_HVoffOvrtmErr_enum : Outport  Port=5
  GbVDP_LeadAcidChgHvOn_flg : Outport  Port=6
  GeVDP_DriveRqst_enum : Outport  Port=7
  GeVDP_ChrgRqst_enum : Outport  Port=8
  GbVDP_2A3Tiout_flg : Outport  Port=9
  GbVDP_2A3ChkSum_flg : Outport  Port=10
  GbVDP_2A3RCMsg_flg : Outport  Port=11
  GbVDP_VCUTiout_flg : Outport  Port=12
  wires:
  GbISP_2A3Tiout_flg/1 -> Relational Operator2/1  "GbISP_2A3Tiout_flg"
  GcISP_ChrgLdReq_numb/1 -> Data Type Conversion7/1  "GcISP_ChrgLdReq_numb"
  GeISP_PreThmVcuPmt_enum/1 -> Data Type Conversion8/1  "GeISP_PreThmVcuPmt_enum"
  GbISP_VcuChrgDisable_flg/1 -> Data Type Conversion9/1  "GbISP_VcuChrgDisable_flg"
  GeISP_HVonOvrtmErr_enum/1 -> Data Type Conversion10/1  "GeISP_HVonOvrtmErr_enum"
  GeISP_HVoffOvrtmErr_enum/1 -> Data Type Conversion11/1  "GeISP_HVoffOvrtmErr_enum"
  GbISP_LeadAcidChgHvOn_flg/1 -> Data Type Conversion12/1  "GbISP_LeadAcidChgHvOn_flg"
  Bus Creator/1 -> Bus Selector/1
  Data Type Conversion7/1 -> Bus Creator/1
  Data Type Conversion8/1 -> Bus Creator/2
  Data Type Conversion9/1 -> Bus Creator/3
  Data Type Conversion10/1 -> Bus Creator/4
  Data Type Conversion11/1 -> Bus Creator/5
  Data Type Conversion12/1 -> Bus Creator/6
  VDP_GcVDP_ChrgLdReq_numb/1 -> GcVDP_ChrgLdReq_numb/1  "GcVDP_ChrgLdReq_numb"
  VDP_GeVDP_PreThmVcuPmt_enum/1 -> GeVDP_PreThmVcuPmt_enum/1  "GeVDP_PreThmVcuPmt_enum"
  VDP_GbVDP_VcuChrgDisable_flg/1 -> GbVDP_VcuChrgDisable_flg/1  "GbVDP_VcuChrgDisable_flg"
  VDP_GeVDP_HVonOvrtmErr_enmu/1 -> GeVDP_HVonOvrtmErr_enum/1  "GeVDP_HVonOvrtmErr_enum"
  VDP_GeVDP_HVoffOvrtmErr_enmu/1 -> GeVDP_HVoffOvrtmErr_enum/1  "GeVDP_HVoffOvrtmErr_enum"
  VDP_GbVDP_LeadAcidChgHvOn_flg/1 -> GbVDP_LeadAcidChgHvOn_flg/1  "GbVDP_LeadAcidChgHvOn_flg"
  Bus Selector/1 -> VDP_GcVDP_ChrgLdReq_numb/1  "<signal1>"
  Bus Selector/2 -> VDP_GeVDP_PreThmVcuPmt_enum/1  "<signal2>"
  Bus Selector/3 -> VDP_GbVDP_VcuChrgDisable_flg/1  "<signal3>"
  Bus Selector/4 -> VDP_GeVDP_HVonOvrtmErr_enmu/1  "<signal4>"
  Bus Selector/5 -> VDP_GeVDP_HVoffOvrtmErr_enmu/1  "<signal5>"
  Switch2/1 -> Unit Delay/1, VDP_GbVDP_LeadAcidChgHvOn_flg/1
  GeISP_VcuPwrReqBatA_enum/1 -> Data Type Conversion15/1  "GeISP_VcuPwrReqBatA_enum"
  VDP_GeVDP_DriveRqst_enum/1 -> GeVDP_DriveRqst_enum/1  "GeVDP_DriveRqst_enum"
  Data Type Conversion15/1 -> VDP_GeVDP_DriveRqst_enum/1, VDP_GeVDP_ChrgRqst_enum/1
  VDP_GeVDP_ChrgRqst_enum/1 -> GeVDP_ChrgRqst_enum/1  "GeVDP_ChrgRqst_enum"
  GbVDP_DiagPermit_flg/1 -> Logical2/2, Logical5/2, Logical4/2
  Constant1/1 -> Relational Operator2/2
  Relational Operator2/1 -> Logical2/1
  Logical2/1 -> GbVDP_2A3Tiout_flgOverWrite/1
  Relational Operator17/1 -> Logical4/1
  Constant2/1 -> Relational Operator17/2
  GbISP_ChkSumMsg2A3Err_flg/1 -> Relational Operator17/1  "GbISP_ChkSumMsg2A3Err_flg"
  Logical4/1 -> VDP_GeVDP_ChrgRqst_enum2/1
  Constant3/1 -> Relational Operator18/2
  Relational Operator18/1 -> Logical5/1
  GbISP_RcMsg2A3Err_flg/1 -> Relational Operator18/1  "GbISP_RcMsg2A3Err_flg"
  Logical5/1 -> VDP_GeVDP_ChrgRqst_enum3/1
  VDP_GeVDP_ChrgRqst_enum2/1 -> GbVDP_2A3ChkSum_flg/1  "GbVDP_2A3ChkSum_flg"
  VDP_GeVDP_ChrgRqst_enum3/1 -> GbVDP_2A3RCMsg_flg/1  "GbVDP_2A3RCMsg_flg"
  GbVDP_2A3Tiout_flgOverWrite/1 -> Relational Operator1/1, GbVDP_2A3Tiout_flg/1  "GbVDP_2A3Tiout_flg"
  Relational Operator1/1 -> Logical1/1
  Constant4/1 -> Relational Operator1/2
  Constant5/1 -> Relational Operator3/2
  Relational Operator3/1 -> Logical1/2
  GbVDP_2A5Tiout_flg/1 -> Relational Operator3/1
  Constant6/1 -> Relational Operator4/2
  GbVDP_2A7Tiout_flg/1 -> Relational Operator4/1
  Relational Operator4/1 -> Logical1/3
  Constant7/1 -> Relational Operator5/2
  GbVDP_0B5Tiout_flg/1 -> Relational Operator5/1
  Logical1/1 -> VDP_GbVDP_VCUTiout_flg/1
  VDP_GbVDP_VCUTiout_flg/1 -> GbVDP_VCUTiout_flg/1  "GbVDP_VCUTiout_flg"
  Relational Operator5/1 -> Logical1/4
  Constant8/1 -> Switch2/1
  Bus Selector/6 -> EdgeRising1/1  "<signal6>"
  EdgeRising1/1 -> Switch2/2
  Unit Delay/1 -> Switch3/3, BMSDelay/1
  Switch3/1 -> Switch2/3
  BMSDelay/1 -> Switch3/2
  Constant9/1 -> Switch3/1
  Constant10/1 -> BMSDelay/2
  Constant11/1 -> BMSDelay/3

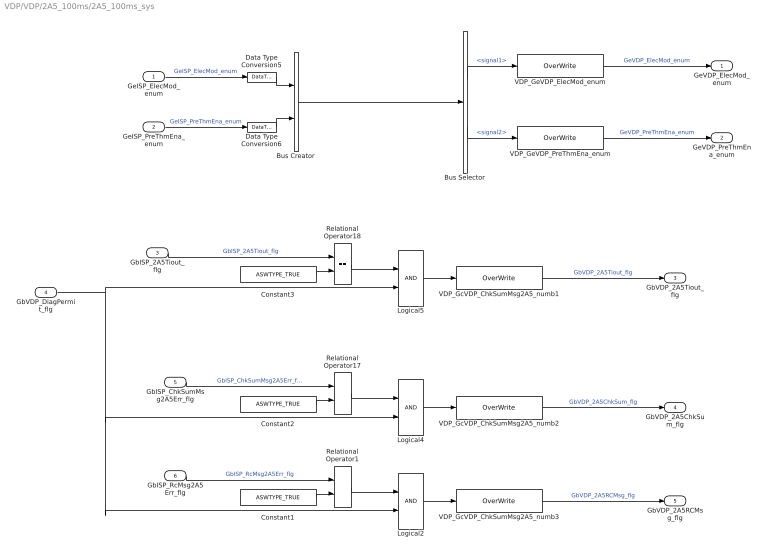
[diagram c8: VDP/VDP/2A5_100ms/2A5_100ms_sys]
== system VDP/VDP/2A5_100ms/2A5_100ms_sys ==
  GeISP_ElecMod_enum : Inport
  GeISP_PreThmEna_enum : Inport  Port=2
  GbISP_2A5Tiout_flg : Inport  Port=3
  GbVDP_DiagPermit_flg : Inport  Port=4
  GbISP_ChkSumMsg2A5Err_flg : Inport  Port=5
  GbISP_RcMsg2A5Err_flg : Inport  Port=6
  Bus Creator : BusCreator  Inputs=2
  Bus Selector : BusSelector  OutputSignals=signal1,signal2
  Constant1 : Constant  Value=ASWTYPE_TRUE
  Constant2 : Constant  Value=ASWTYPE_TRUE
  Constant3 : Constant  Value=ASWTYPE_TRUE
  Data Type Conversion5 : DataTypeConversion
  Data Type Conversion6 : DataTypeConversion
  Logical2 : Logic  OutDataTypeStr=boolean
  Logical4 : Logic  OutDataTypeStr=boolean
  Logical5 : Logic  OutDataTypeStr=boolean
  Relational Operator1 : RelationalOperator  Operator===  OutDataTypeStr=boolean
  Relational Operator17 : RelationalOperator  Operator===  OutDataTypeStr=boolean
  Relational Operator18 : RelationalOperator  Operator===  OutDataTypeStr=boolean
  VDP_GcVDP_ChkSumMsg2A5_numb1 : AIWAYS_Powertrain_BMS_lib/Signals/OverWrite  OverWrite_Value=CbVDP_2A5TioutOvr_flg  OverWrite_flag=CbVDP_2A5TioutOvrSwt_flg
  VDP_GcVDP_ChkSumMsg2A5_numb2 : AIWAYS_Powertrain_BMS_lib/Signals/OverWrite  OverWrite_Value=CbVDP_2A5ChkSumOvr_flg  OverWrite_flag=CbVDP_2A5ChkSumOvrSwt_flg
  VDP_GcVDP_ChkSumMsg2A5_numb3 : AIWAYS_Powertrain_BMS_lib/Signals/OverWrite  OverWrite_Value=CbVDP_2A5RCMsgOvr_flg  OverWrite_flag=CbVDP_2A5RCMsgOvrSwt_flg
  VDP_GeVDP_ElecMod_enum : AIWAYS_Powertrain_BMS_lib/Signals/OverWrite  OverWrite_Value=CeVDP_ElecModOvr_enum  OverWrite_flag=CbVDP_ElecModOvrSwt_flg
  VDP_GeVDP_PreThmEna_enum : AIWAYS_Powertrain_BMS_lib/Signals/OverWrite  OverWrite_Value=CeVDP_PreThmEnaOvr_enum  OverWrite_flag=CbVDP_PreThmEnaOvrSwt_flg
  GeVDP_ElecMod_enum : Outport
  GeVDP_PreThmEna_enum : Outport  Port=2
  GbVDP_2A5Tiout_flg : Outport  Port=3
  GbVDP_2A5ChkSum_flg : Outport  Port=4
  GbVDP_2A5RCMsg_flg : Outport  Port=5
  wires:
  Bus Creator/1 -> Bus Selector/1
  GeISP_ElecMod_enum/1 -> Data Type Conversion5/1  "GeISP_ElecMod_enum"
  GeISP_PreThmEna_enum/1 -> Data Type Conversion6/1  "GeISP_PreThmEna_enum"
  GbISP_2A5Tiout_flg/1 -> Relational Operator18/1  "GbISP_2A5Tiout_flg"
  Bus Selector/1 -> VDP_GeVDP_ElecMod_enum/1  "<signal1>"
  Bus Selector/2 -> VDP_GeVDP_PreThmEna_enum/1  "<signal2>"
  VDP_GeVDP_ElecMod_enum/1 -> GeVDP_ElecMod_enum/1  "GeVDP_ElecMod_enum"
  VDP_GeVDP_PreThmEna_enum/1 -> GeVDP_PreThmEna_enum/1  "GeVDP_PreThmEna_enum"
  Data Type Conversion5/1 -> Bus Creator/1
  Data Type Conversion6/1 -> Bus Creator/2
  Constant3/1 -> Relational Operator18/2
  Relational Operator18/1 -> Logical5/1
  Logical5/1 -> VDP_GcVDP_ChkSumMsg2A5_numb1/1
  GbISP_RcMsg2A5Err_flg/1 -> Relational Operator1/1  "GbISP_RcMsg2A5Err_flg"
  Constant1/1 -> Relational Operator1/2
  Relational Operator1/1 -> Logical2/1
  Logical2/1 -> VDP_GcVDP_ChkSumMsg2A5_numb3/1
  Logical4/1 -> VDP_GcVDP_ChkSumMsg2A5_numb2/1
  GbVDP_DiagPermit_flg/1 -> Logical4/2, Logical2/2, Logical5/2
  GbISP_ChkSumMsg2A5Err_flg/1 -> Relational Operator17/1  "GbISP_ChkSumMsg2A5Err_flg"
  Constant2/1 -> Relational Operator17/2
  Relational Operator17/1 -> Logical4/1
  VDP_GcVDP_ChkSumMsg2A5_numb1/1 -> GbVDP_2A5Tiout_flg/1  "GbVDP_2A5Tiout_flg"
  VDP_GcVDP_ChkSumMsg2A5_numb2/1 -> GbVDP_2A5ChkSum_flg/1  "GbVDP_2A5ChkSum_flg"
  VDP_GcVDP_ChkSumMsg2A5_numb3/1 -> GbVDP_2A5RCMsg_flg/1  "GbVDP_2A5RCMsg_flg"

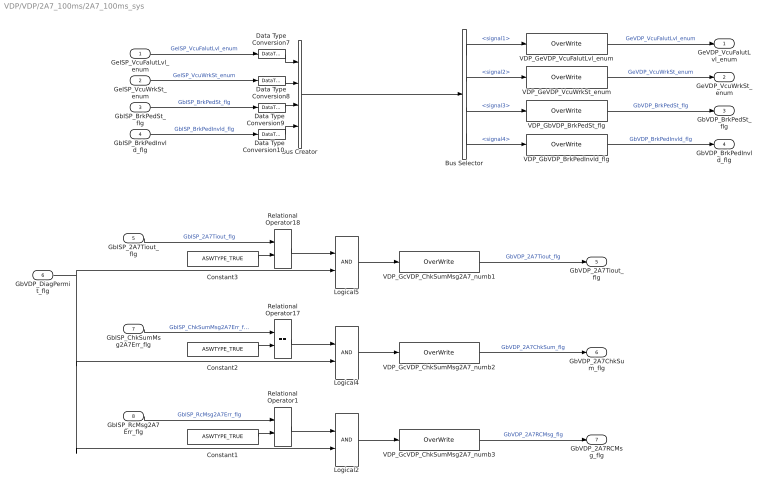
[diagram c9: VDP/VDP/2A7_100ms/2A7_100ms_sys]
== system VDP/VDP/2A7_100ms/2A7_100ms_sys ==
  GeISP_VcuFalutLvl_enum : Inport
  GeISP_VcuWrkSt_enum : Inport  Port=2
  GbISP_BrkPedSt_flg : Inport  Port=3
  GbISP_BrkPedInvld_flg : Inport  Port=4
  GbISP_2A7Tiout_flg : Inport  Port=5
  GbVDP_DiagPermit_flg : Inport  Port=6
  GbISP_ChkSumMsg2A7Err_flg : Inport  Port=7
  GbISP_RcMsg2A7Err_flg : Inport  Port=8
  Bus Creator : BusCreator  Inputs=4
  Bus Selector : BusSelector  OutputSignals=signal1,signal2,signal3,signal4
  Constant1 : Constant  Value=ASWTYPE_TRUE
  Constant2 : Constant  Value=ASWTYPE_TRUE
  Constant3 : Constant  Value=ASWTYPE_TRUE
  Data Type Conversion{7..10} (4 alike) : DataTypeConversion
  Logical2 : Logic  OutDataTypeStr=boolean
  Logical4 : Logic  OutDataTypeStr=boolean
  Logical5 : Logic  OutDataTypeStr=boolean
  Relational Operator1 : RelationalOperator  Operator===  OutDataTypeStr=boolean
  Relational Operator17 : RelationalOperator  Operator===  OutDataTypeStr=boolean
  Relational Operator18 : RelationalOperator  Operator===  OutDataTypeStr=boolean
  VDP_GbVDP_BrkPedInvld_flg : AIWAYS_Powertrain_BMS_lib/Signals/OverWrite  OverWrite_Value=CbVDP_BrkPedInvldOvr_flg  OverWrite_flag=CbVDP_BrkPedInvldOvrSwt_flg
  VDP_GbVDP_BrkPedSt_flg : AIWAYS_Powertrain_BMS_lib/Signals/OverWrite  OverWrite_Value=CbVDP_BrkPedStOvr_flg  OverWrite_flag=CbVDP_BrkPedStOvrSwt_flg
  VDP_GcVDP_ChkSumMsg2A7_numb1 : AIWAYS_Powertrain_BMS_lib/Signals/OverWrite  OverWrite_Value=CbVDP_2A7TioutOvr_flg  OverWrite_flag=CbVDP_2A7TioutOvrSwt_flg
  VDP_GcVDP_ChkSumMsg2A7_numb2 : AIWAYS_Powertrain_BMS_lib/Signals/OverWrite  OverWrite_Value=CbVDP_2A7ChkSumOvr_flg  OverWrite_flag=CbVDP_2A7ChkSumOvrSwt_flg
  VDP_GcVDP_ChkSumMsg2A7_numb3 : AIWAYS_Powertrain_BMS_lib/Signals/OverWrite  OverWrite_Value=CbVDP_2A7RCMsgOvr_flg  OverWrite_flag=CbVDP_2A7RCMsgOvrSwt_flg
  VDP_GeVDP_VcuFalutLvl_enum : AIWAYS_Powertrain_BMS_lib/Signals/OverWrite  OverWrite_Value=CeVDP_VcuFalutLvlOvr_enum  OverWrite_flag=CbVDP_VcuFalutLvlOvrSwt_flg
  VDP_GeVDP_VcuWrkSt_enum : AIWAYS_Powertrain_BMS_lib/Signals/OverWrite  OverWrite_Value=CeVDP_VcuWrkStOvr_enum  OverWrite_flag=CbVDP_VcuWrkStOvrSwt_flg
  GeVDP_VcuFalutLvl_enum : Outport
  GeVDP_VcuWrkSt_enum : Outport  Port=2
  GbVDP_BrkPedSt_flg : Outport  Port=3
  GbVDP_BrkPedInvld_flg : Outport  Port=4
  GbVDP_2A7Tiout_flg : Outport  Port=5
  GbVDP_2A7ChkSum_flg : Outport  Port=6
  GbVDP_2A7RCMsg_flg : Outport  Port=7
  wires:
  Bus Creator/1 -> Bus Selector/1
  GeISP_VcuFalutLvl_enum/1 -> Data Type Conversion7/1  "GeISP_VcuFalutLvl_enum"
  GeISP_VcuWrkSt_enum/1 -> Data Type Conversion8/1  "GeISP_VcuWrkSt_enum"
  GbISP_BrkPedSt_flg/1 -> Data Type Conversion9/1  "GbISP_BrkPedSt_flg"
  GbISP_BrkPedInvld_flg/1 -> Data Type Conversion10/1  "GbISP_BrkPedInvld_flg"
  GbISP_2A7Tiout_flg/1 -> Relational Operator18/1  "GbISP_2A7Tiout_flg"
  VDP_GeVDP_VcuFalutLvl_enum/1 -> GeVDP_VcuFalutLvl_enum/1  "GeVDP_VcuFalutLvl_enum"
  VDP_GeVDP_VcuWrkSt_enum/1 -> GeVDP_VcuWrkSt_enum/1  "GeVDP_VcuWrkSt_enum"
  VDP_GbVDP_BrkPedSt_flg/1 -> GbVDP_BrkPedSt_flg/1  "GbVDP_BrkPedSt_flg"
  VDP_GbVDP_BrkPedInvld_flg/1 -> GbVDP_BrkPedInvld_flg/1  "GbVDP_BrkPedInvld_flg"
  Bus Selector/1 -> VDP_GeVDP_VcuFalutLvl_enum/1  "<signal1>"
  Bus Selector/2 -> VDP_GeVDP_VcuWrkSt_enum/1  "<signal2>"
  Bus Selector/3 -> VDP_GbVDP_BrkPedSt_flg/1  "<signal3>"
  Bus Selector/4 -> VDP_GbVDP_BrkPedInvld_flg/1  "<signal4>"
  Data Type Conversion7/1 -> Bus Creator/1
  Data Type Conversion8/1 -> Bus Creator/2
  Data Type Conversion9/1 -> Bus Creator/3
  Data Type Conversion10/1 -> Bus Creator/4
  Constant3/1 -> Relational Operator18/2
  Logical5/1 -> VDP_GcVDP_ChkSumMsg2A7_numb1/1
  GbVDP_DiagPermit_flg/1 -> Logical5/2, Logical4/2, Logical2/2
  Constant1/1 -> Relational Operator1/2
  Logical4/1 -> VDP_GcVDP_ChkSumMsg2A7_numb2/1
  GbISP_ChkSumMsg2A7Err_flg/1 -> Relational Operator17/1  "GbISP_ChkSumMsg2A7Err_flg"
  Constant2/1 -> Relational Operator17/2
  Relational Operator1/1 -> Logical2/1
  GbISP_RcMsg2A7Err_flg/1 -> Relational Operator1/1  "GbISP_RcMsg2A7Err_flg"
  Relational Operator17/1 -> Logical4/1
  Logical2/1 -> VDP_GcVDP_ChkSumMsg2A7_numb3/1
  Relational Operator18/1 -> Logical5/1
  VDP_GcVDP_ChkSumMsg2A7_numb1/1 -> GbVDP_2A7Tiout_flg/1  "GbVDP_2A7Tiout_flg"
  VDP_GcVDP_ChkSumMsg2A7_numb2/1 -> GbVDP_2A7ChkSum_flg/1  "GbVDP_2A7ChkSum_flg"
  VDP_GcVDP_ChkSumMsg2A7_numb3/1 -> GbVDP_2A7RCMsg_flg/1  "GbVDP_2A7RCMsg_flg"

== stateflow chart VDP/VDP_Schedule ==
  (default) -> (junction 50)
  (junction 50) -> (junction 13) : { VDP_0B5_10ms; VDP_2A3_10ms; }
  (junction 13) -> (junction 150) : { TimeCounter100ms ++; }
  (junction 150) -> (junction 503) : [TimeCounter100ms >= Const100ms]
  (junction 150) -> (junction 505)
  (junction 503) -> (junction 505) : {VDP_2A5_100ms; VDP_2A7_100ms; TimeCounter100ms = 0; }
  data: Const100ms constant uint8 =10; TimeCounter100ms local uint8
  events: output FUNCTION_CALL_EVENT; output FUNCTION_CALL_EVENT; output FUNCTION_CALL_EVENT; output FUNCTION_CALL_EVENT
